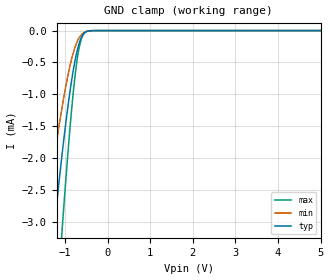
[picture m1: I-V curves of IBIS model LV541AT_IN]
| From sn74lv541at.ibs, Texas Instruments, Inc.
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[Model]   LV541AT_IN
Model_type  Input
Vinl=0.8
Vinh=2.0
| variable   typ   min   max
C_comp   1.01pF   0.86pF   1.12pF
[Temperature Range]   40   100   -40
| Ambient temperature   25   85   -40
[Voltage range]   5   4.5   5.5
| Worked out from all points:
|   GND clamp passes 1 mA (typ) near -0.89 V on its own axis
[GND Clamp]
| LV541AT_IN
|   Voltage   I(typ)   I(min)   I(max)
-5.5V     -44.86mA   -30.18mA   -56.6mA
-1.52V    -5.002mA   -3.26mA    -7.744mA
-1.465V   -4.59mA    -2.984mA   -7.149mA
-1.265V   -3.175mA   -2.032mA   -5.049mA
-1.085V   -2.032mA   -1.263mA   -3.277mA
-1.06V    -1.885mA   -1.164mA   -3.043mA
-910mV    -1.078mA   -632.4uA   -1.732mA
-825mV    -695.5uA   -392.8uA   -1.092mA
-750mV    -419.2uA   -231.1uA   -624.4uA
-640mV    -144.7uA   -83.96uA   -183.2uA
-530mV    -29.42uA   -20.61uA   -28.33uA
5V        17.64nA    1.142nA    163.4nA
